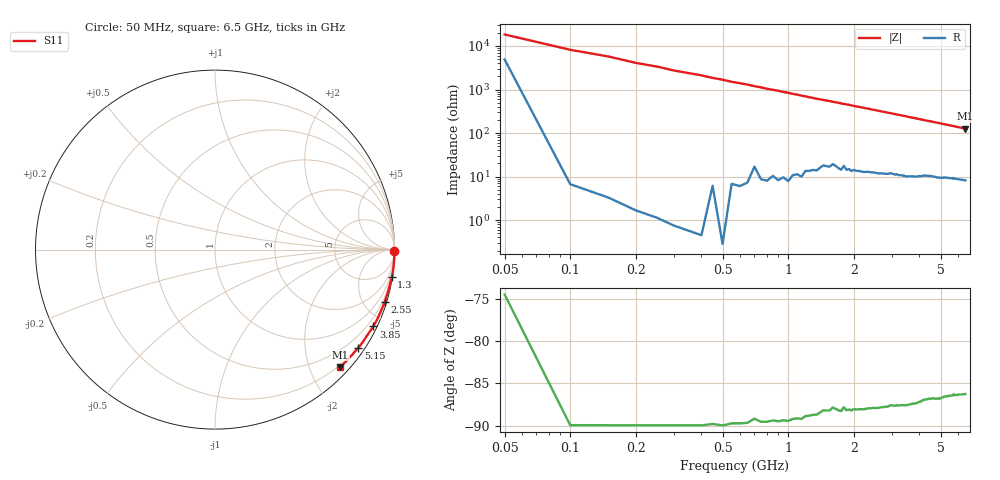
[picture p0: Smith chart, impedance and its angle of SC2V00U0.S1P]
! Infineon Technologies  Discrete & RF Semiconductors
! BAR63-02L
! Si PIN Diode in TSLP-2
! VR = 2 V
! S-Parameters:  March  2002
# GHz  S  MA  R  50
!  f  S11
! GHz  MAG  ANG
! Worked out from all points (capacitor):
!   130 points, 50 MHz to 6.5 GHz, reference 50 ohm
!   read as one part to ground: C = 185 fF near 50 MHz
!   lowest |Z| = 126 ohm at 6.5 GHz (marker M1)
!   S11 on the Smith chart (normalised r, x): 50 MHz: open; 1.3 GHz: 0, -13; 2.55 GHz: 0.24, -6.60; 3.85 GHz: 0.20, -4.34; 5.15 GHz: 0.19, -3.22; 6.5 GHz: 0.16, -2.52
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0.05  0.9986 -0.3
0.1  1 -0.7
0.3  1 -2.1
0.4  1 -2.7
0.55  0.9997 -3.8
0.9  0.9991 -6.1
1.3  0.9966 -8.9
1.35  0.9964 -9.3
1.55  0.9943 -10.5
1.6  0.993 -10.9
1.7  0.9937 -11.5
1.75  0.9938 -11.9
1.9  0.9926 -12.8
2.05  0.9921 -13.9
2.5  0.9896 -16.8
2.55  0.9894 -17.2
3.3  0.9843 -22.1
3.85  0.98 -25.9
4.1  0.9768 -27.5
4.9  0.97 -32.7
5.15  0.9676 -34.4
5.35  0.965 -35.6
5.4  0.9652 -36.0
5.7  0.9627 -37.9
5.75  0.9607 -38.1
5.8  0.9614 -38.6
5.95  0.9606 -39.5
6.5  0.9565 -43.1
